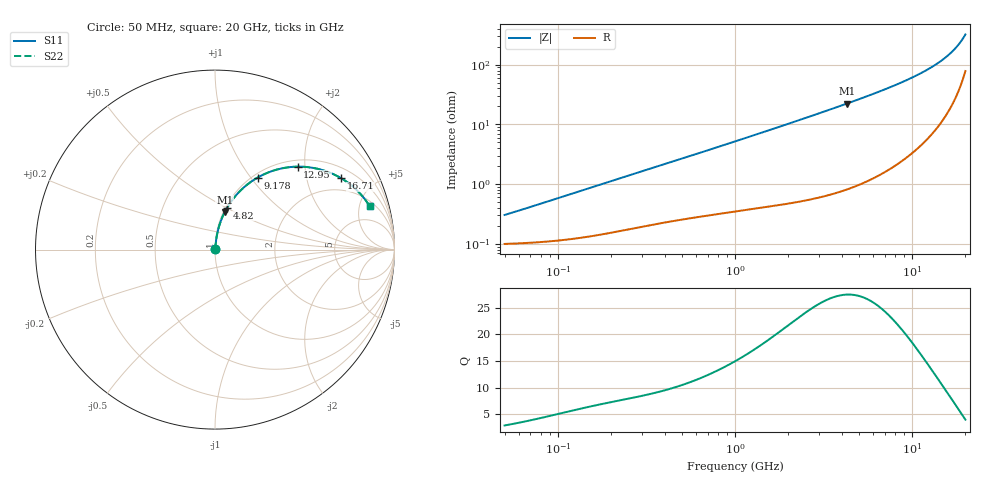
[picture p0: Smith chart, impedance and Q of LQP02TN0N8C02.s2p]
!Murata Part Number: LQP02TN0N8C02
!These Parameters are Measured in Series Mode Connection
!  o--[Z]--o
!Port1  Port2
!  o-------o
!Freq. Start=50[MHz] Stop=20[GHz], 401[Steps]
# Hz S RI R 50
!Freq.(Hz) S11(Real) S11(Imag) S21(Real) S21(Imag) S12(Real) S12(Imag) S22(Real) S22(Imag)
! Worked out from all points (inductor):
!   401 points, 50 MHz to 20 GHz, reference 50 ohm
!   read as one part in series: L = 912 pH near 52.3 MHz
!   highest Q = 27.5 at 4.276 GHz (marker M1), where L = 829 pH
!   S11 on the Smith chart (normalised r, x): 50 MHz: 1.00, +0.01; 4.82 GHz: 1.02, +0.51; 9.178 GHz: 1.05, +1.08; 12.95 GHz: 1.14, +1.83; 16.71 GHz: 1.41, +3.22; 20 GHz: 2.57, +6.24
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5e7  0.001 0.00287  0.999 -0.00287  0.999 -0.00287  0.001 0.00287
6.646115e7  0.00104 0.0038  0.999 -0.0038  0.999 -0.0038  0.00104 0.0038
1.364002e8  0.00132 0.0077  0.9987 -0.0077  0.9987 -0.0077  0.00132 0.0077
3.721004e8  0.00258 0.02  0.9974 -0.02  0.9974 -0.02  0.00258 0.02
1e9  0.00609 0.0513  0.9939 -0.0513  0.9939 -0.0513  0.00609 0.0513
1.714689e9  0.0119 0.0864  0.9881 -0.0864  0.9881 -0.0864  0.0119 0.0864
2.728004e9  0.0245 0.1357  0.9755 -0.1357  0.9755 -0.1357  0.0245 0.1357
4.275624e9  0.0542 0.209  0.9458 -0.209  0.9458 -0.209  0.0542 0.209
4.81993e9  0.0679 0.2339  0.9321 -0.2339  0.9321 -0.2339  0.0679 0.2339
6.125241e9  0.1074 0.2909  0.8926 -0.2909  0.8926 -0.2909  0.1074 0.2909
7.442007e9  0.1572 0.3433  0.8428 -0.3433  0.8428 -0.3433  0.1572 0.3433
9.178299e9  0.2376 0.4014  0.7624 -0.4014  0.7624 -0.4014  0.2376 0.4014
1.098561e10  0.3377 0.4438  0.6623 -0.4438  0.6623 -0.4438  0.3377 0.4438
1.295331e10  0.4609 0.4622  0.5391 -0.4622  0.5391 -0.4622  0.4609 0.4622
1.396067e10  0.5271 0.4583  0.4729 -0.4583  0.4729 -0.4583  0.5271 0.4583
1.482269e10  0.5838 0.4473  0.4162 -0.4473  0.4162 -0.4473  0.5838 0.4473
1.573793e10  0.6427 0.4277  0.3573 -0.4277  0.3573 -0.4277  0.6427 0.4277
1.670968e10  0.7024 0.398  0.2976 -0.398  0.2976 -0.398  0.7024 0.398
1.800918e10  0.7747 0.3454  0.2253 -0.3454  0.2253 -0.3454  0.7747 0.3454
1.88369e10  0.8148 0.3051  0.1852 -0.3051  0.1852 -0.3051  0.8148 0.3051
1.940974e10  0.8394 0.2747  0.1606 -0.2747  0.1606 -0.2747  0.8394 0.2747
2e10  0.8618 0.2416  0.1382 -0.2416  0.1382 -0.2416  0.8618 0.2416
